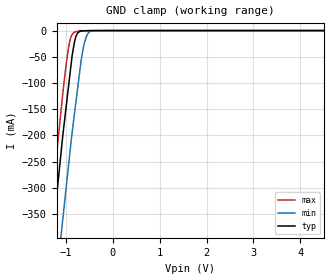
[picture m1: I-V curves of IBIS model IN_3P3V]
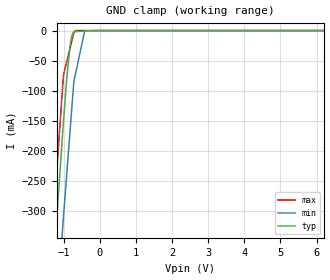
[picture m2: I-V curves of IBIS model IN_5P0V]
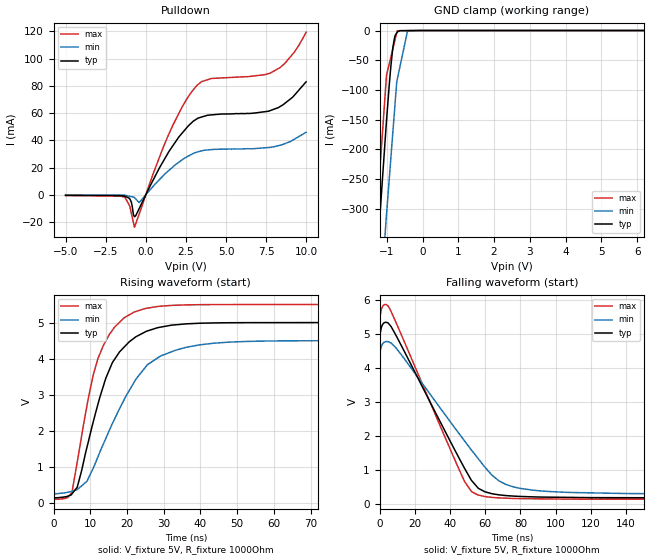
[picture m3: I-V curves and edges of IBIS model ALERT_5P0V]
| Texas Instruments Incorporated
| Digital Temperature Sensor and Thermal Watchdog With Two-Wire Interface
| Marketing part#   Voltage Range   Package-type   #pins/pkg drawing
| LM75AD   2.7V - 5.5V   SOIC   8-pin D
| LM75ADGK   2.7V - 5.5V   VSSOP   8-pin DGK
[IBIS Ver]   4.1
[File name]   lm75a.ibs
[File Rev]   1.0
[Date]   04/14/2015
[Source]   Model built from spectre simulations at:
   Texas Instruments Incorporated.
   Webench Design Center
   12500 TI Blvd
   Dallas, TX -75243
   For Support e-mail: elab_ibis@list.ti.com
[Notes]   Revision History
   Rev 1.0: 04/14/2015
   - Non monotonic behavior result of circuit behavior
   - ccomp values are based on PVT settings:
   MIN: Low Voltage, High Temperature, Weak Process
   TYP: Nominal Voltage, Nominal Temperature, Nominal Process
   MAX: High Voltage, Low Temperature, Fast Process
   - C_comp although listed in numerical order of value are obtained from varying PVT conditions.
   For PVT conditions for each specific value, refer to the buffer description under respective [Model].
   IBIS model user is responsible for using appropriate C_comp to simulate for Signal Integrity.
[Disclaimer]  This model is designed as an aid for customers of Texas Instruments
 TI and its licensors and suppliers make no warranties, either expressed
 or implied, with respect to this  model, including the warranties of
 merchantability or fitness for a particular purpose.
 The model is provided solely on an "as is" basis. The entire risk as to
 its quality and performance is with the customer.
[Copyright] (C)Copyright 2015 Texas Instruments Incorporated.
   All rights reserved.
[Component]   LM75AD
[Manufacturer]  Texas Instruments Incorporated
[Package]   |8-pin SOIC D package
|   typ   min   max
R_pkg   0.07717   0.00230   0.11690
L_pkg   2.32134nH   1.36253nH   2.80112nH
C_pkg   0.39851pF   0.31326pF   0.46592pF
[Pin]   signal_name   model_name   R_pin   L_pin   C_pin
1   SDA   SDA   0.11215   2.70023n   0.38408p
2   SCL   IN   0.03900   2.09764n   0.46592p
3   OS   ALERT   0.02513   1.85198n   0.46577p
4   GND   GND   0.11876   2.80112n   0.38992p
5   A2   IN   0.00230   1.36253n   0.31326p
6   A1   IN   0.11690   2.72346n   0.40067p
7   A0   IN   0.09586   2.40528n   0.38694p
8   VCC   POWER   0.10729   2.62852n   0.38154p
[Component]   LM75ADGK
[Manufacturer]  Texas Instruments Incorporated
[Package]   |8-pin VSSP DGK package
|   typ   min   max
R_pkg   2.900e-02   1.000e-03   3.800e-02
L_pkg   1.570e-09   9.040e-10   1.800e-0
C_pkg   2.930e-13   2.360e-13   3.130e-1
[Pin]   signal_name   model_name   R_pin   L_pin   C_pin
1   SDA   SDA   1.000e-03   9.040e-10   2.360e-13
2   SCL   IN   3.000e-02   1.598e-09   3.100e-13
3   OS   ALERT   3.000e-02   1.607e-09   3.130e-13
4   GND   GND   3.600e-02   1.760e-09   2.880e-13
5   A2   IN   3.800e-02   1.800e-09   2.900e-13
6   A1   IN   3.000e-02   1.606e-09   3.120e-13
7   A0   IN   3.000e-02   1.596e-09   3.120e-13
8   VCC   POWER   3.300e-02   1.687e-09   2.830e-13
[Model Selector] IN
IN_3P3V   3.3V INPUT
IN_5P0V   5.0V INPUT
[Model Selector] ALERT
ALERT_3P3V   3.3V OPEN DRAIN OUTPUT
ALERT_5P0V   5.0V OPEN DRAIN OUTPUT
[Model Selector] SDA
SDA_3P3V   3.3V OPEN DRAIN I/O
SDA_5P0V   5.0V OPEN DRAIN I/O
| Models and submodels in the file (6): IN_3P3V (Input), IN_5P0V (Input), ALERT_5P0V (Open_drain), ALERT_3P3V (Open_drain), SDA_5P0V (I/O_open_drain), SDA_3P3V (I/O_open_drain)
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|   Model IN_3P3V
[Model]   IN_3P3V
Model_type   Input
Vinl = .99
Vinh = 2.31
|   typ   min   max
|   (nom PVT)   (fast PVT)   (slow PVT)
C_comp   0.397p   0.367p   0.437p
| Where   nom PVT is  Nominal Process, 3.3V, 27C
|   Fast PVT is Strong Process, 3.6V, -40C
|   Slow PVT is Weak Process, 2.7V, 150C
[Model spec]
|subparameter
Vinl   0.99   0.81   1.08
Vinh   2.31   1.89   2.52
[Voltage Range]   3.3   2.7   3.6
[Temperature Range]   27   150   -40
[Power Clamp Reference]   3.3   2.7   3.6
[GND Clamp Reference]   0   0   0
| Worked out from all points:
|   GND clamp passes 1 mA (typ) near -0.68 V on its own axis
[GND Clamp]
|   Voltage   I(typ)   I(min)   I(max)
-3.3V     -2.267A    -2.366A    -2.221A
-1.457V   -549.7mA   -703.3mA   -471.5mA
-1.271V   -380.8mA   -538mA     -300.3mA
-1.073V   -206.5mA   -365.5mA   -126.6mA
-937.3mV  -101.3mA   -252mA     -29.02mA
-867.1mV  -47.5mA    -194.4mA   -7.696mA
-807.5mV  -18.37mA   -151.6mA   -2.602mA
-743.3mV  -3.966mA   -105.5mA   -1.239mA
-627.9mV  -557uA     -32.47mA   -240uA
-553.7mV  -210uA     -9.056mA   -322.9uA
-454.7mV  0A         -1.134mA   -210.5uA
6.59V     0A         0A         0A
|   Model IN_5P0V
[Model]   IN_5P0V
Model_type   Input
Vinl = 1.5
Vinh = 3.5
|   typ   min   max
|   (nom PVT)   (fast PVT)   (slow PVT)
C_comp   0.364p   0.338p   0.390p
| Where   nom PVT is  Nominal Process, 5.0V, 27C
|   Fast PVT is Strong Process, 4.5V, -40C
|   Slow PVT is Weak Process, 5.5V, 150C
[Model spec]
|subparameter
Vinl   1.5   1.35   1.65
Vinh   3.5   3.15   3.85
[Voltage Range]   5   4.5   5.5
[Temperature Range]   27   150   -40
[Power Clamp Reference]   5   4.5   5.5
[GND Clamp Reference]   0   0   0
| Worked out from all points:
|   GND clamp passes 1 mA (typ) near -0.46 V on its own axis
[GND Clamp]
|   Voltage   I(typ)   I(min)   I(max)
-5V       -3.854A    -3.901A    -3.837A
-1.307V   -413mA     -569.8mA   -332.8mA
-1.021V   -162.3mA   -320.5mA   -85.1mA
-1.007V   -151mA     -309.8mA   -73.39mA
-938.8mV  -96.77mA   -256.2mA   -56.91mA
-901.3mV  -69.8mA    -226.8mA   -47.86mA
-826.3mV  -25.46mA   -168mA     -29.76mA
-770mV    -7.609mA   -123.9mA   -16.19mA
-720.7mV  -2.395mA   -85.11mA   -4.278mA
-707.1mV  -1.7mA     -81.31mA   -1.012mA
-420.7mV  -903.3uA   -758.2uA   0A
9.985V    0A         0A         0A
|   Model ALERT_5P0V
[Model]   ALERT_5P0V
Model_type   Open_drain
Polarity   Non-Inverting
Vmeas = 2.5
Vref = 5
Cref = 15pF
Rref = 1000
|   typ   min   max
|   (nom PVT)   (fast PVT)   (slow PVT)
C_comp   0.526p   0.482p   0.579p
|C_comp (ON state)   0.526p   0.482p   0.579p
|C_comp (OFF state)   0.624p   0.613p   0.652p
| Where   nom PVT is  Nominal Process, 5.0V, 27C
|   Fast PVT is Strong Process, 4.5V, -40C
|   Slow PVT is Weak Process, 5.5V, 150C
[Voltage Range]   5   4.5   5.5
[Temperature Range]   27   150   -40
[Pullup Reference]   5   4.5   5.5
[Pulldown Reference]   0   0   0
[Power Clamp Reference]   5   4.5   5.5
[GND Clamp Reference]   0   0   0
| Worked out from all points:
|   slope of the pulldown table from 0 to 0.75 V, typ, clamps not added: 42.9 ohm
|   GND clamp passes 1 mA (typ) near -0.66 V on its own axis
|   falling waveform, V_fixture 5V, R_fixture 1000Ohm: 20-80 % time 28.7ns typ, 36.3ns min, 26.6ns max; typ from 5 V to 0.191 V
|   rising waveform, V_fixture 5V, R_fixture 1000Ohm: 20-80 % time 8.78ns typ, 12.7ns min, 7.33ns max; typ from 0.19 V to 5 V
[Pulldown]
|   Voltage   I(typ)   I(min)   I(max)
-5V       -417.2uA   -165.8uA   -573.8uA
-1.307V   -1.051mA   -358.2uA   -1.762mA
-901.3mV  -5.416mA   -1.411mA   -13.66mA
-707.1mV  -16.16mA   -2.055mA   -23.79mA
-420.7mV  -10.34mA   -5.763mA   -14.46mA
1.378V    30.51mA    17.27mA    43.12mA
2.278V    45.5mA     25.77mA    64.87mA
3.178V    55.73mA    31.3mA     80.25mA
4.078V    58.66mA    33.15mA    85.39mA
7.753V    61.84mA    34.81mA    89.36mA
8.653V    67.08mA    37.53mA    96.39mA
9.985V    82.98mA    45.92mA    119.3mA
[GND Clamp]
|   Voltage   I(typ)   I(min)   I(max)
-5V       -3.855A    -3.902A    -3.838A
-1.314V   -419.6mA   -576.2mA   -339.7mA
-1.307V   -413.8mA   -570.4mA   -333.5mA
-1.021V   -163.5mA   -321.3mA   -87.03mA
-1.007V   -152.2mA   -310.7mA   -75.38mA
-901.3mV  -71.49mA   -227.9mA   -48.94mA
-845mV    -36.99mA   -183.9mA   -34.89mA
-770mV    -9.358mA   -125.2mA   -16.15mA
-720.7mV  -4.046mA   -86.54mA   -3.813mA
-707.1mV  -2.713mA   -82.69mA   -431.6uA
-420.7mV  -190.2uA   -1.157mA   -98.59uA
9.985V    0A         0A         0A
[Ramp]
R_load = 1000
|   typ   min   max
dV/dt_r   2.88584/8.78003e-09   2.51962/1.26739e-08   3.21037/7.31644e-09
dV/dt_f   2.88532/2.87259e-08   2.51725/3.62427e-08   3.2102/2.65671e-08
[Falling Waveform]
V_fixture = 5V
V_fixture_min = 4.5V
V_fixture_max = 5.5V
R_fixture = 1000Ohm
C_fixture = 0F
|   Time   V(typ)   V(min)   V(max)
0s        5V         4.5V       5.5V
2.034ns   5.308V     4.736V     5.842V
3.813ns   5.348V     4.784V     5.872V
5.959ns   5.26V      4.755V     5.728V
44.3ns    1.442V     2.137V     1.123V
52.3ns    698.2mV    1.589V     371.8mV
59.77ns   371.8mV    1.096V     231.4mV
67.72ns   281.7mV    693.1mV    192.2mV
79.72ns   234.8mV    472.2mV    170.6mV
199.9ns   191.1mV    304.6mV    149.7mV
[Rising Waveform]
V_fixture = 5V
V_fixture_min = 4.5V
V_fixture_max = 5.5V
R_fixture = 1000Ohm
C_fixture = 0F
|   Time   V(typ)   V(min)   V(max)
0s        190.2mV    300.6mV    149.3mV
5.015ns   259.1mV    329.7mV    301.6mV
6.461ns   445mV      380.6mV    1.146V
10.8ns    2.25V      972.2mV    3.549V
13.55ns   3.24V      1.638V     4.362V
17.99ns   4.192V     2.62V      5.01V
24.99ns   4.744V     3.761V     5.39V
33.13ns   4.937V     4.231V     5.479V
47.72ns   4.995V     4.458V     5.498V
199.9ns   5V         4.5V       5.5V
